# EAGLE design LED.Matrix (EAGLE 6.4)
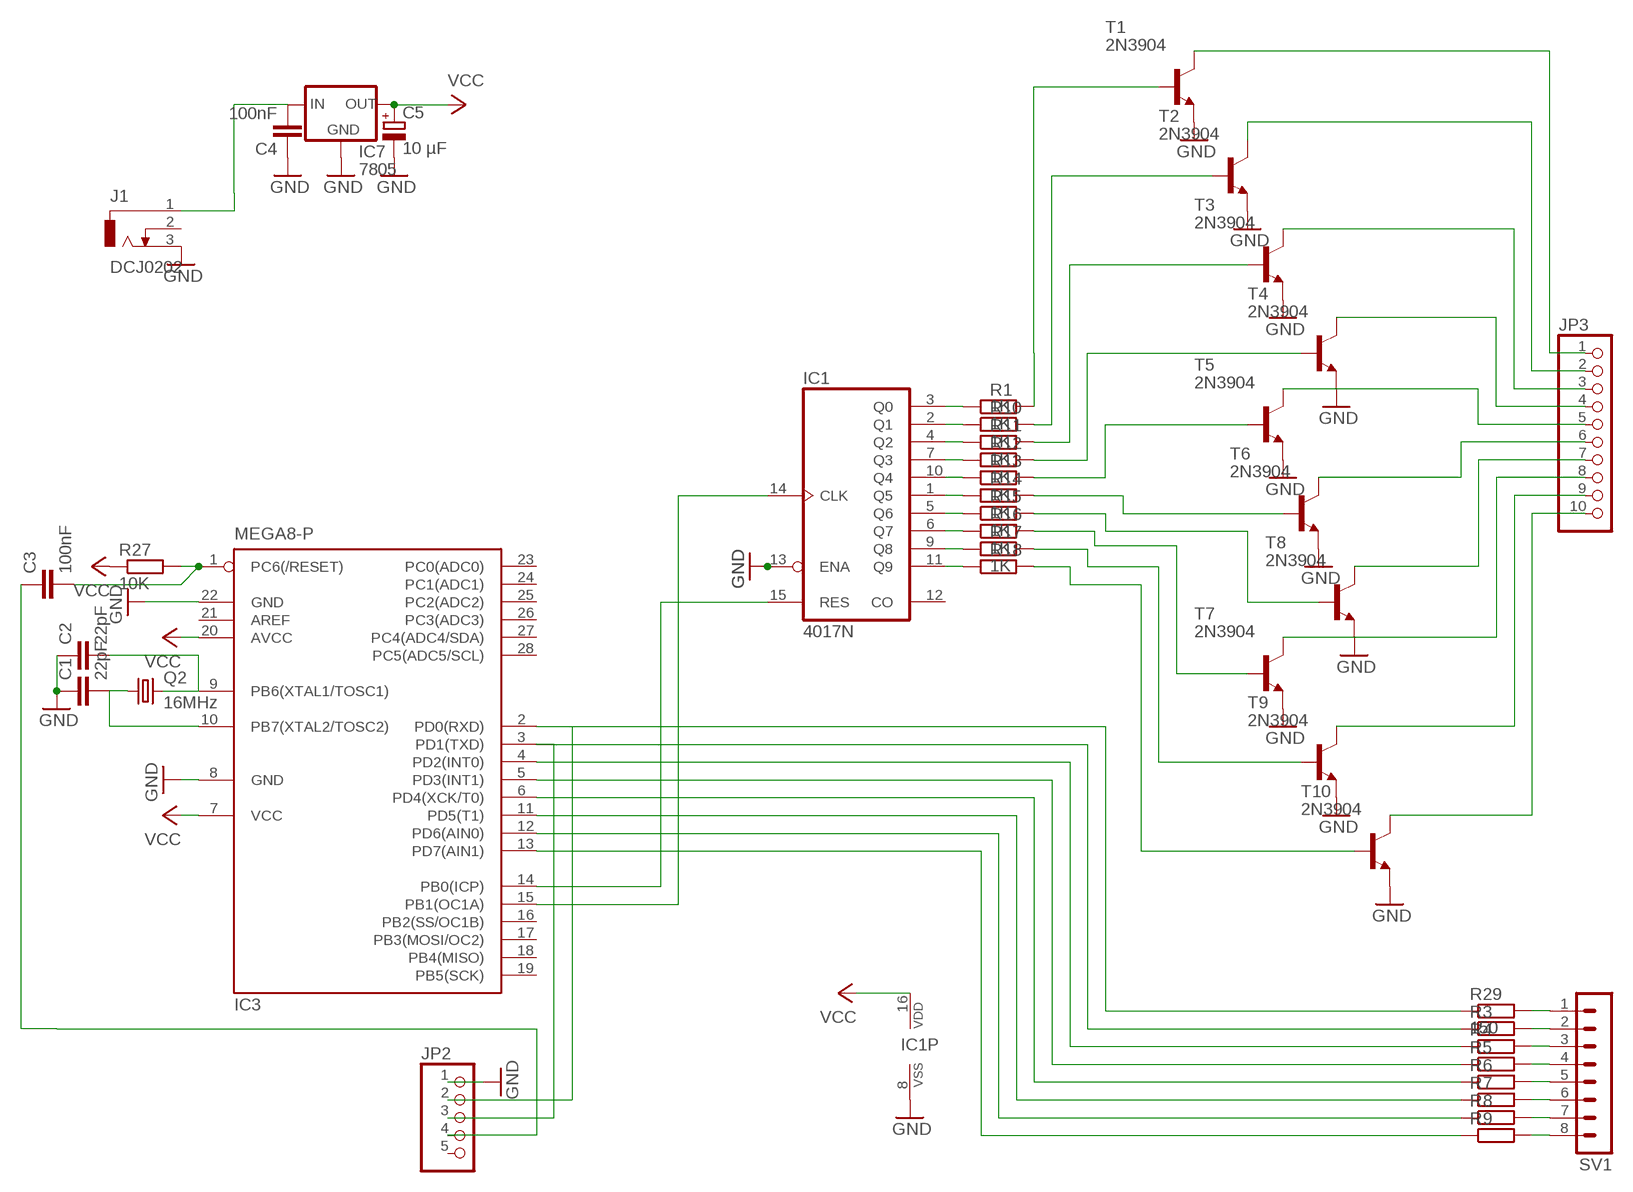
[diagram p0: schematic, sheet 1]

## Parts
C1  22pF  C-EU025-030X050  [C025-030X050]
C2  22pF  C-EU025-030X050  [C025-030X050]
C3  100nF  C-EU025-030X050  [C025-030X050]
C4  100nF  C-EU025-030X050  [C025-030X050]
C5  10 µF  CPOL-EUB45181B  [B45181B]
IC1  4017N  [DIL16]
IC3  MEGA8-P  [DIL28-3]
IC7  7805  V_REG_78XXSIDE  [78XXL]
J1  DCJ0202  [DCJ0202]
JP2  PINHD-1X5  [1X05]
JP3  PINHD-1X10  [1X10]
Q2  16MHz  CRYSTALHC49S  [HC49/S]
R1  1K  R-EU_0207/7  [0207/7]
R3  R-EU_0207/7  [0207/7]
R4  R-EU_0207/7  [0207/7]
R5  R-EU_0207/7  [0207/7]
R6  R-EU_0207/7  [0207/7]
R7  R-EU_0207/7  [0207/7]
R8  R-EU_0207/7  [0207/7]
R9  R-EU_0207/7  [0207/7]
R10  1K  R-EU_0207/7  [0207/7]
R11  1K  R-EU_0207/7  [0207/7]
R12  1K  R-EU_0207/7  [0207/7]
R13  1K  R-EU_0207/7  [0207/7]
R14  1K  R-EU_0207/7  [0207/7]
R15  1K  R-EU_0207/7  [0207/7]
R16  1K  R-EU_0207/7  [0207/7]
R17  1K  R-EU_0207/7  [0207/7]
R18  1K  R-EU_0207/7  [0207/7]
R27  10K  R-EU_0207/7  [0207/7]
R29  150  R-EU_0207/7  [0207/7]
SV1  MA08-1  [MA08-1]
T1  2N3904  [TO92]
T2  2N3904  [TO92]
T3  2N3904  [TO92]
T4  2N3904  [TO92]
T5  2N3904  [TO92]
T6  2N3904  [TO92]
T7  2N3904  [TO92]
T8  2N3904  [TO92]
T9  2N3904  [TO92]
T10  2N3904  [TO92]

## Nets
GND [GND]: C1.1 C2.1 C4.1 C5.- IC1.8(VSS) IC1.13(ENA) IC3.8(GND) IC3.22(GND) IC7.GND J1.3 JP2.1 T1.3(E) T2.3(E) T3.3(E) T4.3(E) T5.3(E) T6.3(E) T7.3(E) T8.3(E) T9.3(E) T10.3(E)
N$1: IC1.15(RES) IC3.14(PB0(ICP))
N$2: C3.1 JP2.4
N$3: IC1.14(CLK) IC3.15(PB1(OC1A))
N$4: R29.2 SV1.1
N$5: IC1.3(Q0) R1.1
N$6: R3.2 SV1.2
N$7: R1.2 T1.2(B)
N$8: R4.2 SV1.3
N$9: IC1.2(Q1) R10.1
N$10: R5.2 SV1.4
N$11: IC1.4(Q2) R11.1
N$12: R7.2 SV1.6
N$13: IC1.7(Q3) R12.1
N$14: R6.2 SV1.5
N$15: IC1.10(Q4) R13.1
N$16: R8.2 SV1.7
N$17: IC1.1(Q5) R14.1
N$18: R9.2 SV1.8
N$19: IC1.5(Q6) R15.1
N$22: IC3.4(PD2(INT0)) R4.1
N$23: IC3.5(PD3(INT1)) R5.1
N$24: IC3.6(PD4(XCK/T0)) R6.1
N$25: IC3.11(PD5(T1)) R7.1
N$26: IC3.12(PD6(AIN0)) R8.1
N$27: IC3.13(PD7(AIN1)) R9.1
N$28: IC1.6(Q7) R16.1
N$29: IC1.9(Q8) R17.1
N$30: IC1.11(Q9) R18.1
N$31: R10.2 T2.2(B)
N$32: R11.2 T3.2(B)
N$33: R12.2 T4.2(B)
N$34: R13.2 T5.2(B)
N$35: R14.2 T6.2(B)
N$36: R15.2 T8.2(B)
N$37: R16.2 T7.2(B)
N$38: R17.2 T9.2(B)
N$39: R18.2 T10.2(B)
N$40: JP3.1 T1.1(C)
N$41: JP3.2 T2.1(C)
N$42: JP3.3 T3.1(C)
N$43: JP3.4 T4.1(C)
N$44: JP3.5 T5.1(C)
N$45: JP3.6 T6.1(C)
N$46: JP3.7 T8.1(C)
N$47: JP3.8 T7.1(C)
N$48: JP3.9 T9.1(C)
N$49: JP3.10 T10.1(C)
N$59: IC3.3(PD1(TXD)) JP2.3 R3.1
N$81: C3.2 IC3.1(PC6(/RESET)) R27.2
N$82: C2.2 IC3.9(PB6(XTAL1/TOSC1)) Q2.2
N$83: C1.2 IC3.10(PB7(XTAL2/TOSC2)) Q2.1
N$84: IC3.2(PD0(RXD)) JP2.2 R29.1
N$86: C4.2 IC7.IN J1.1
VCC [VCC]: C5.+ IC1.16(VDD) IC3.7(VCC) IC3.20(AVCC) IC7.OUT R27.1
Unconnected: IC1.12(CO) IC3.16(PB2(SS/OC1B)) IC3.17(PB3(MOSI/OC2)) IC3.18(PB4(MISO)) IC3.19(PB5(SCK)) IC3.21(AREF) IC3.23(PC0(ADC0)) IC3.24(PC1(ADC1)) IC3.25(PC2(ADC2)) IC3.26(PC3(ADC3)) IC3.27(PC4(ADC4/SDA)) IC3.28(PC5(ADC5/SCL)) J1.2 JP2.5

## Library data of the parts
C1-C4 = resistor:C-EU: CAPACITOR, European symbol
C5 = resistor:CPOL-EU: POLARIZED CAPACITOR, European symbol
IC1 = 40xx:4017: COUNTER/DIVIDER
IC3 = atmel:MEGA8-P: MICROCONTROLLER 8 Kbytes FLASH, 1 kbytes SRAM, 512 bytes EEPROM, USART, 4-channel 10 bit ADC, 2-channel 8 bit ADC Pin compatible with Atmega48, ATMega88, ATMega168 Source: avr.lbr; OC_FARNELL: unknown; OC_NEWARK: unknown
IC7 = SparkFun:V_REG_78XX: Voltage Regulator Standard 7805 5V regulator. IGO (Input Ground Output). Spark Fun Electronics SKU : COM-00107
J1 = con-jack:DCJ0202: DC POWER JACK Source: DCJ0202.pdf; OC_FARNELL: unknown; OC_NEWARK: unknown
JP2 = pinhead:PINHD-1X5: PIN HEADER
JP3 = pinhead:PINHD-1X10: PIN HEADER
Q2 = crystal:CRYSTAL: CRYSTAL; OC_FARNELL: 1667008; OC_NEWARK: unknown
R1 R3-R18 R27 R29 = resistor:R-EU_: RESISTOR, European symbol
SV1 = con-lstb:MA08-1: PIN HEADER; OC_FARNELL: unknown; OC_NEWARK: unknown
T1-T10 = transistor:2N3904: NPN TRANSISTOR

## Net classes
1 VCC: width 0.508 mm
2 GND: width 0.508 mm

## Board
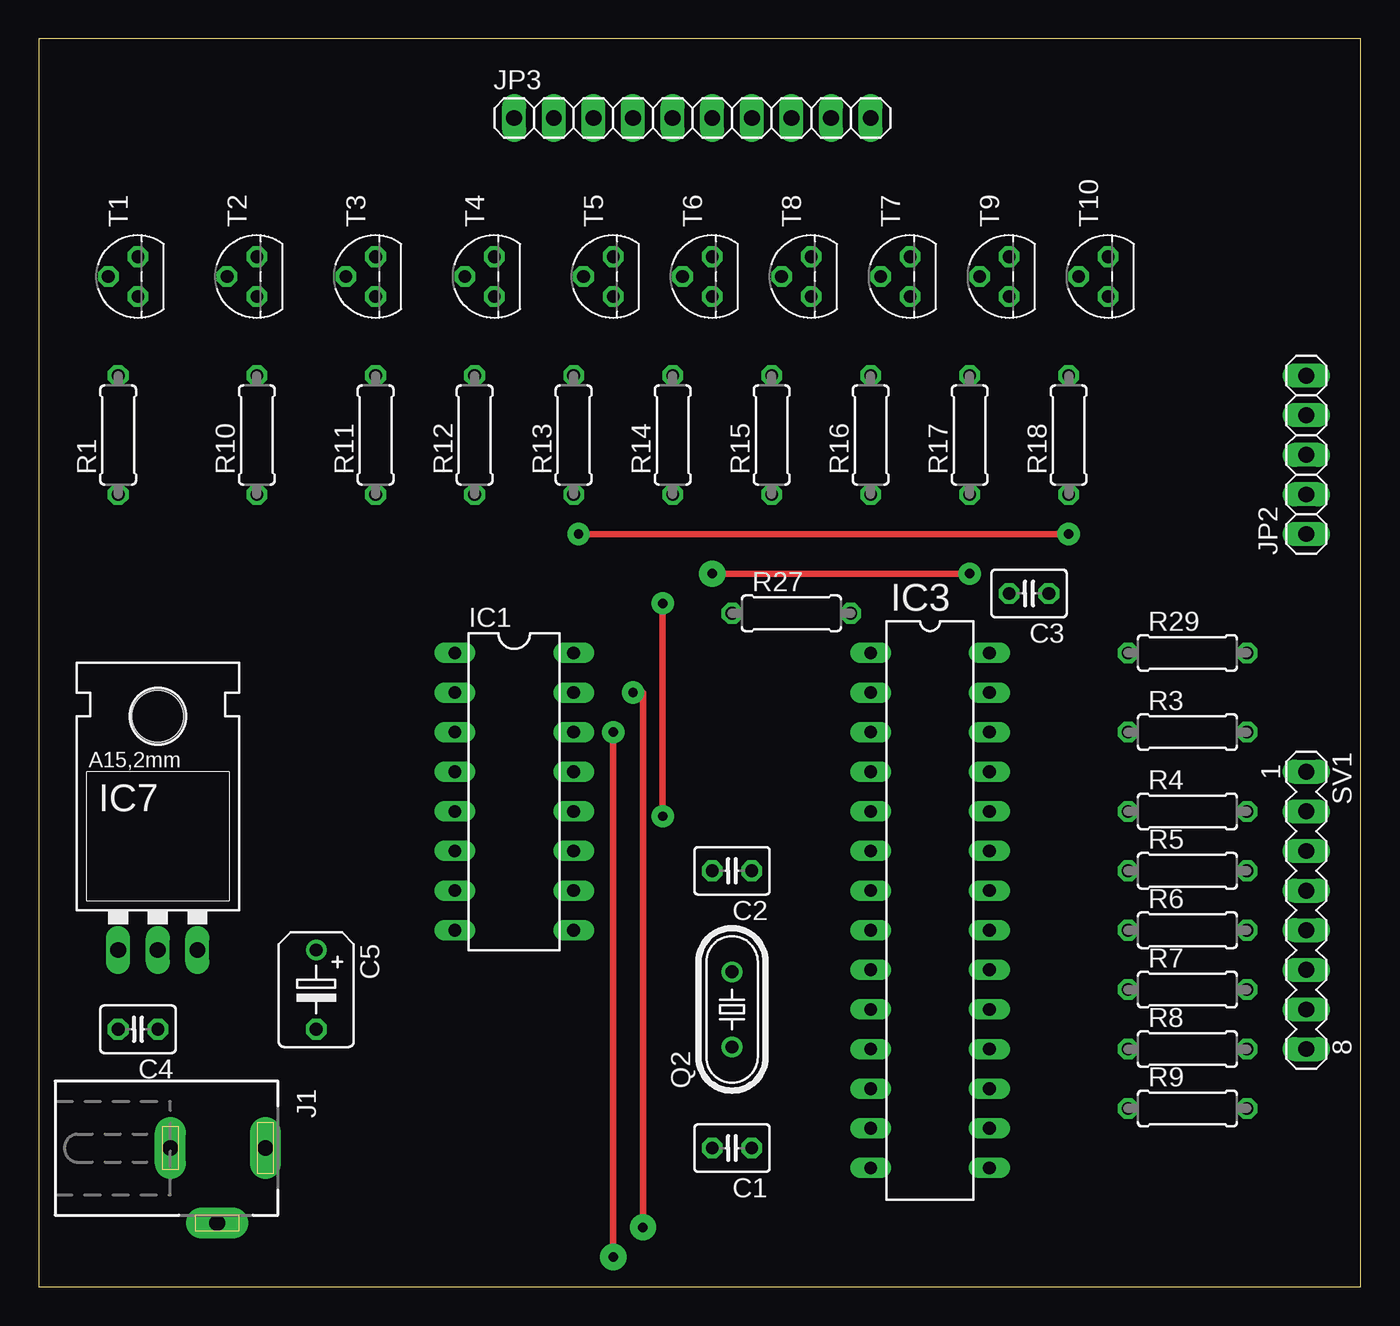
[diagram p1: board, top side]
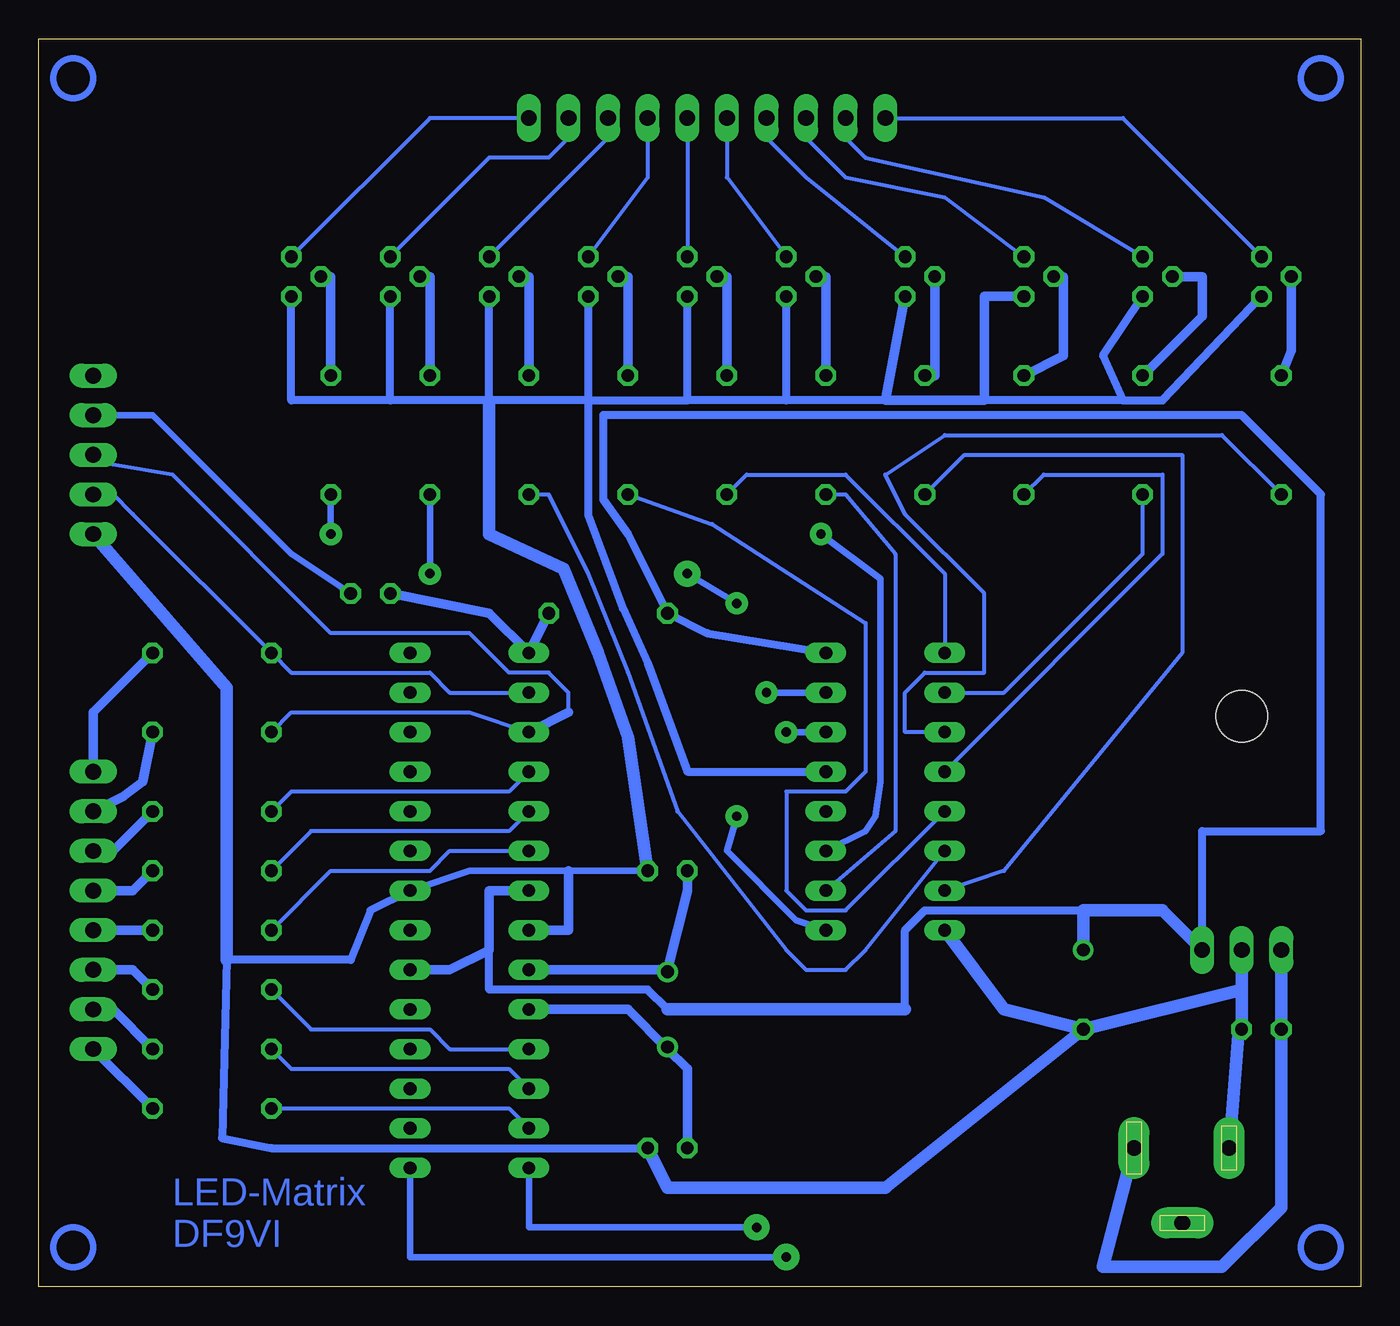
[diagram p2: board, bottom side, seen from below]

Size 84.76 x 80 mm. Coordinates in mm from the lower left corner, seen from the top.
Outline: 0,0 84.76,0 84.76,80 0,80 0,0
Copper layers (1*16): Top 0.035mm / dielectric 1.5mm / Bottom 0.035mm
Design rules "default *": minimum track width 10mil, minimum drill 24mil, track to track 10mil, track to pad 10mil, pad to pad 8mil, via to via 8mil, smd to smd 8mil, copper to edge 40mil, drill to drill 8mil, minimum pad ring 10mil, minimum via ring 8mil, stop-mask expansion 4mil, vias tented up to drill 0mil, thermal gap 10mil

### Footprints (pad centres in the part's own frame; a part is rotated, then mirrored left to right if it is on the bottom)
C025-030X050 = drill 0.813 octagon: 1 -1.27,0; 2 1.27,0
B45181B = drill 0.813: + -2.54,0 | drill 0.813 octagon: - 2.54,0
DIL16 = drill 0.813 long: 1 -8.89,-3.81; 2 -6.35,-3.81; 3 -3.81,-3.81; 4 -1.27,-3.81; 5 1.27,-3.81; 6 3.81,-3.81; 7 6.35,-3.81; 8 8.89,-3.81; 9 8.89,3.81; 10 6.35,3.81; 11 3.81,3.81; 12 1.27,3.81; 13 -1.27,3.81; 14 -3.81,3.81; 15 -6.35,3.81; 16 -8.89,3.81
DIL28-3 = drill 0.813 long: 1 -16.51,-3.81; 2 -13.97,-3.81; 3 -11.43,-3.81; 4 -8.89,-3.81; 5 -6.35,-3.81; 6 -3.81,-3.81; 7 -1.27,-3.81; 8 1.27,-3.81; 9 3.81,-3.81; 10 6.35,-3.81; 11 8.89,-3.81; 12 11.43,-3.81; 13 13.97,-3.81; 14 16.51,-3.81; 15 16.51,3.81; 16 13.97,3.81; 17 11.43,3.81; 18 8.89,3.81; 19 6.35,3.81; 20 3.81,3.81; 21 1.27,3.81; 22 -1.27,3.81; 23 -3.81,3.81; 24 -6.35,3.81; 25 -8.89,3.81; 26 -11.43,3.81; 27 -13.97,3.81; 28 -16.51,3.81
78XXL = drill 1.016 long: GND 0,-3.81; IN -2.54,-3.81; OUT 2.54,-3.81 | hole 3.302: 0,11.176
DCJ0202 = drill 1 pad 2 long: 1 0,3.1; 2 4.8,0; 3 0,-3
1X05 = drill 1.016 long: 1 -5.08,0; 2 -2.54,0; 3 0,0; 4 2.54,0; 5 5.08,0
1X10 = drill 1.016 long: 1 -11.43,0; 2 -8.89,0; 3 -6.35,0; 4 -3.81,0; 5 -1.27,0; 6 1.27,0; 7 3.81,0; 8 6.35,0; 9 8.89,0; 10 11.43,0
HC49/S = drill 0.813: 1 -2.413,0; 2 2.413,0
0207/7 = drill 0.813 octagon: 1 -3.81,0; 2 3.81,0
MA08-1 = drill 1.016 long: 1 -8.89,0; 2 -6.35,0; 3 -3.81,0; 4 -1.27,0; 5 1.27,0; 6 3.81,0; 7 6.35,0; 8 8.89,0
TO92 = drill 0.813 octagon: 1 1.27,0; 2 0,1.905; 3 -1.27,0

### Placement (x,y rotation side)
C1  44.45,8.89 180 top
C2  44.45,26.67 180 top
C3  63.5,44.45 180 top
C4  6.35,16.51 180 top
C5  17.78,19.05 270 top
IC1  30.48,31.75 270 top
IC3  57.15,24.13 270 top
IC7  7.62,25.4 0 top
J1  11.43,8.89 270 top
JP2  81.28,53.34 90 top
JP3  41.91,74.93 0 top
Q2  44.45,17.78 90 top
R1  5.08,54.61 90 top
R3  73.66,35.56 0 top
R4  73.66,30.48 0 top
R5  73.66,26.67 0 top
R6  73.66,22.86 0 top
R7  73.66,19.05 0 top
R8  73.66,15.24 0 top
R9  73.66,11.43 0 top
R10  13.97,54.61 90 top
R11  21.59,54.61 90 top
R12  27.94,54.61 90 top
R13  34.29,54.61 90 top
R14  40.64,54.61 90 top
R15  46.99,54.61 90 top
R16  53.34,54.61 90 top
R17  59.69,54.61 90 top
R18  66.04,54.61 90 top
R27  48.26,43.18 0 top
R29  73.66,40.64 0 top
SV1  81.28,24.13 270 top
T1  6.35,64.77 90 top
T2  13.97,64.77 90 top
T3  21.59,64.77 90 top
T4  29.21,64.77 90 top
T5  36.83,64.77 90 top
T6  43.18,64.77 90 top
T7  55.88,64.77 90 top
T8  49.53,64.77 90 top
T9  62.23,64.77 90 top
T10  68.58,64.77 90 top

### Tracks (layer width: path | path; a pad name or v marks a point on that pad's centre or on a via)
GND
  Bottom 0.406: 50.8,26.67 C2.1 57.15,26.67 IC3.22 | C4.1 7.79,16.51
  Bottom 0.508: T1.3 12.7,56.83 15.24,56.83 | 15.24,56.83 16.51,59.69 T2.3 | 30.48,56.83 T4.3 | 15.24,56.83 24.13,56.83 30.48,56.83 | 36.83,56.83 T5.3 | 30.48,56.83 36.83,56.83 | 43.18,56.83 43.18,60.96 | 43.18,60.96 T6.3 43.18,60.96 | 36.83,56.83 43.18,56.83 | IC1.13 43.18,33.02 45.72,40.01 47.31,43.5 49.53,49.53 49.53,56.83 | T8.3 49.53,56.83 | 55.88,56.83 T7.3 | 49.53,56.83 55.88,56.83 | 62.23,56.83 T9.3 | 55.88,56.83 62.23,56.83 | T10.3 68.58,56.83 62.23,56.83 | 43.18,56.83 43.18,60.96 | 49.53,56.83 43.18,56.83 | IC3.22 63.5,24.13 64.77,20.95 72.71,20.95 73.02,9.53 69.85,8.89 C1.1
  Bottom 0.61: T3.3 24.13,63.5 24.13,56.83 30.48,56.83 T4.3 | 50.8,26.67 50.8,22.86 IC3.8
  Bottom 0.813: C1.1 44.45,6.35 30.48,6.35 C5.- | IC7.GND 7.62,19.05 | 7.62,19.05 C4.1 | IC1.8 22.86,17.78 C5.- | 7.62,19.05 C5.- | JP2.1 72.71,38.42 72.71,20.95 | 7.79,16.51 J1.3 | C2.1 46.99,35.24 48.9,40.64 51.12,46.04 55.88,48.26 55.88,56.83
N$1  (via drill 0.6 pad 1.42, 0.6 pad 1.68)
  Top 0.406: v38.1,38.1 38.73,38.1 v38.73,3.81
  Bottom 0.406: IC1.15 v38.1,38.1 | v38.73,3.81 53.34,3.81 IC3.14
N$2
  Bottom 0.406: C3.1 68.58,46.99 74.93,53.34 77.47,55.88 JP2.4
N$3  (via drill 0.6 pad 1.42, 0.6 pad 1.68)
  Top 0.406: v36.83,35.56 v36.83,1.91
  Bottom 0.406: IC1.14 v36.83,35.56 | v36.83,1.91 60.96,1.91 60.96,3.81 IC3.15
N$4
  Bottom 0.61: R29.2 81.28,36.83 SV1.1
N$5
  Bottom 0.254: R1.1 8.89,54.61 26.67,54.61 30.48,52.07 29.21,49.53 24.13,44.45 24.13,39.37 27.94,39.37 29.21,38.1 29.21,35.56 IC1.3
N$6
  Bottom 0.61: R3.2 78.1,32.38 79.38,31.43 SV1.2
N$7
  Bottom 0.61: R1.2 4.44,60.01 T1.2
N$8
  Bottom 0.254: SV1.3 80.01,27.94
  Bottom 0.61: 80.01,27.94 R4.2
N$9
  Bottom 0.254: R10.1 13.97,46.99 22.86,38.1 IC1.2
N$10
  Bottom 0.61: R5.2 78.74,25.4 SV1.4
N$11
  Bottom 0.254: IC1.4 12.7,46.99 12.7,52.07 20.32,52.07 R11.1
N$12
  Bottom 0.61: R7.2 78.74,20.32 SV1.6
N$13
  Bottom 0.254: IC1.7 22.86,26.67 11.43,40.64 11.43,53.34 25.4,53.34 R12.1
N$14
  Bottom 0.61: SV1.5 R6.2
N$15
  Bottom 0.254: IC1.10 29.85,29.21 29.85,46.99 33.02,50.8 R13.1
N$16
  Bottom 0.254: SV1.7 80.01,17.78
  Bottom 0.61: 80.01,17.78 R8.2
N$17
  Bottom 0.254: IC1.1 26.67,45.72 33.02,52.07 39.37,52.07 R14.1
N$18
  Bottom 0.61: SV1.8 R9.2
N$19
  Bottom 0.254: IC1.5 33.02,24.13 35.56,24.13 36.83,25.4 36.83,31.75 33.02,31.75 31.75,33.02 31.75,42.55 41.59,48.9 R15.1
N$22
  Bottom 0.254: R4.1 68.58,31.75 54.61,31.75 IC3.4
N$23
  Bottom 0.254: R5.1 67.31,29.21 54.61,29.21 IC3.5
N$24
  Bottom 0.254: IC3.6 58.42,27.94 59.69,26.67 66.04,26.67 R6.1
N$25
  Bottom 0.254: IC3.11 58.42,15.24 59.69,16.51 67.31,16.51 R7.1
N$26
  Bottom 0.254: IC3.12 54.61,13.97 68.58,13.97 R8.1
N$27
  Bottom 0.254: IC3.13 54.61,11.43 R9.1
N$28
  Bottom 0.254: IC1.6 31.75,21.59 33.02,20.32 35.56,20.32 36.83,21.59 43.82,30.48 46.99,39.37 49.53,45.72 52.07,50.8 R16.1
N$29  (via drill 0.6 pad 1.42, 0.6 pad 1.68)
  Top 0.406: v40.01,43.81 v40.01,30.16 | v43.18,45.72 45.72,45.72 v59.69,45.72
  Bottom 0.406: v43.18,45.72 v40.01,43.81 | v40.01,30.16 40.64,27.94 36.2,23.5 IC1.9 | v59.69,45.72 R17.1
N$30  (via drill 0.6 pad 1.42)
  Top 0.406: v34.61,48.26 v66.04,48.26
  Bottom 0.406: IC1.11 31.75,29.21 31.11,30.16 30.8,32.38 30.8,45.4 v34.61,48.26 | v66.04,48.26 R18.1
N$31
  Bottom 0.254: 11.43,64.77 T2.2
  Bottom 0.61: R10.2 10.16,62.23 10.16,64.77 11.43,64.77
N$32
  Bottom 0.61: R11.2 19.05,59.69 19.05,63.5 19.05,64.77 T3.2
N$33
  Bottom 0.61: R12.2 27.3,58.42 27.3,59.05 27.3,63.82 T4.2
N$34
  Bottom 0.61: R13.2 34.29,64.77 T5.2
N$35
  Bottom 0.61: R14.2 40.64,64.77 T6.2
N$36
  Bottom 0.61: R15.2 46.99,64.77 T8.2
N$37
  Bottom 0.61: R16.2 53.34,64.77 T7.2
N$38
  Bottom 0.61: R17.2 59.69,64.77 T9.2
N$39
  Bottom 0.61: R18.2 66.04,64.77 T10.2
N$40
  Bottom 0.254: T1.1 15.24,74.93 JP3.1
N$41
  Bottom 0.254: T2.1 20.32,69.85 31.75,72.39 33.02,73.66 JP3.2
N$42
  Bottom 0.254: T3.1 26.67,69.85 33.02,71.12 35.56,73.66 JP3.3
N$43
  Bottom 0.254: T4.1 35.56,71.12 36.83,72.39 38.1,73.66 JP3.4
N$44
  Bottom 0.254: T5.1 40.64,71.12 JP3.5
N$45
  Bottom 0.254: JP3.6 T6.1
N$46
  Bottom 0.254: T8.1 45.72,71.12 45.72,73.66 JP3.7
N$47
  Bottom 0.254: T7.1 48.26,73.66 JP3.8
N$48
  Bottom 0.254: T9.1 55.88,72.39 52.07,72.39 50.8,73.66 JP3.9
N$49
  Bottom 0.254: T10.1 59.69,74.93 JP3.10
N$59
  Bottom 0.254: IC3.3 57.15,36.83 68.58,36.83 R3.1 | JP2.3 80.01,52.7 76.2,52.07 66.04,41.91 57.15,41.91 54.61,39.37 52.07,39.37 50.8,38.1 50.8,36.83
  Bottom 0.61: 50.8,36.83 IC3.3
N$81
  Bottom 0.61: C3.2 55.88,43.18 IC3.1 R27.2
N$82
  Bottom 0.254: 44.45,20.32 Q2.2 44.45,20.32
  Bottom 0.61: C2.2 43.18,25.4 44.45,20.32 IC3.9
N$83
  Bottom 0.254: 44.45,15.24 Q2.1 44.45,15.24
  Bottom 0.61: C1.2 43.18,13.97 44.45,15.24 46.99,17.78 IC3.10
N$84
  Bottom 0.254: IC3.2 58.42,38.1 59.69,39.37 68.58,39.37 R29.1 78.74,49.53 80.01,50.8 JP2.2
N$86
  Bottom 0.813: IC7.IN C4.2 5.08,13.97 5.08,12.7 5.08,5.08 8.89,1.27 16.51,1.27 J1.1
VCC
  Bottom 0.508: IC1.16 41.91,41.91 R27.1 46.99,48.26 48.58,50.48 48.58,55.88 7.62,55.88 2.54,50.8 2.54,29.21 10.16,29.21 IC7.OUT | 17.78,24.13 27.94,24.13 29.21,22.86 29.21,17.78 | 55.88,21.59 55.88,19.05 45.72,19.05 44.45,17.78
  Bottom 0.61: IC3.20 58.42,20.32 55.88,21.59 55.88,25.4 IC3.7
  Bottom 0.813: IC7.OUT 12.7,24.13 17.78,24.13 C5.+ | 29.21,17.78 44.45,17.78
(copper drawn outside any net)
  shapes: Bottom circle x4

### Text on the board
Bottom: LED-Matrix / DF9VI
